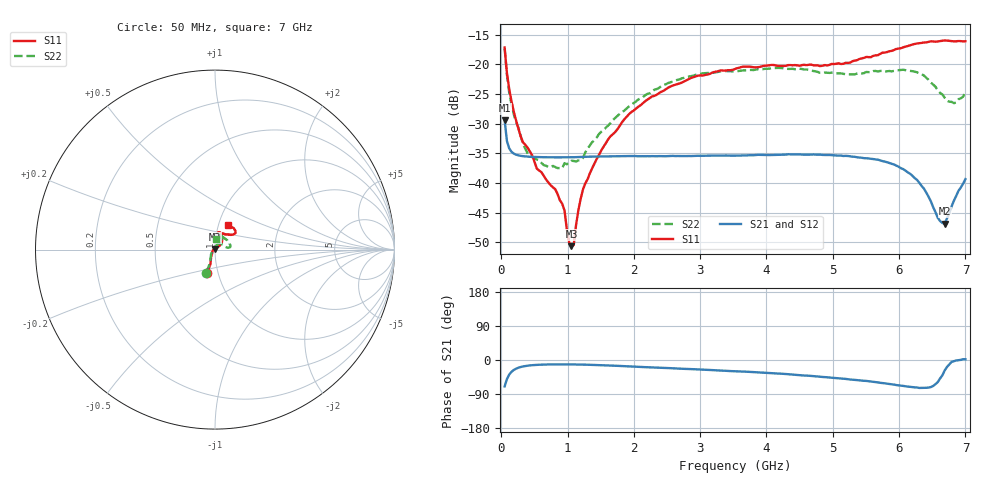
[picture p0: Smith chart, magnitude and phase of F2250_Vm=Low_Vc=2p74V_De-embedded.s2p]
! Integrated Device Technology
! Corporate Headquarters
! 6024 Silver Creek Valley Road
! San Jose, CA 95138  USA
! Phone:  1-408-284-8200
! Toll Free:  1-800-223-1366
! Webpage:  http://www.idt.com/
! Timing and RF Division
! 515 Groton Road, Suite 102
! Westford, MA 01886-6024
! Device:  F2250
! Description: Voltage Variable RF Attenuator
! Frequency:  50.0 -  6000.00 MHz
! Package:  3x3 mm Thin QFN Plastic Package: 16 pin
! Ports:  2 RF, 3 DC
!  Pin  1  = GND
!  Pin  2  = NC
!  Pin  3  = RF1  = Port 1
!  Pin  4  = NC
!  Pin  5  = GND
!  Pin  6  = GND
!  Pin  7  = GND
!  Pin  8  = GND
!  Pin  9  = NC
!  Pin 10  = RF2  = Port 2
!  Pin 11  = NC
!  Pin 12  = GND
!  Pin 13  = GND
!  Pin 14  = VCNTRL
!  Pin 15  = VDD
!  Pin 16  = VMODE
! Vcntrl:  2.740 Volts
! Vmode:  +0.000 Volts
! Vdd:  +3.30  Volts
! Current:  1.174 mA
! Data:  The device was measured on a the F2250 evaluation board which has
!  individual transmission lines to the RF pins.  Data was collected
!  using a calibrated network analyzer.  The evaluation board was
!  de-embedded using a TRL calibration technique.
!  The reference plane is the edge of the package pin.
! Misc:  SN 10
!  Action Tracker AT0258
! Date Measured:  2014-11-26
! Date:  2015-10-15  MJV
! Note:
!  Integrated Device Technology supplies this data as a sample of measured
!  data at the package pin for this product.  Your particular data for this
!  product may vary.
!  Data was taken at 25 degrees C.
!  Integrated Device Technology reserves the right to change this data at anytime.
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# GHz S dB R 50
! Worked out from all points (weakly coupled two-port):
!   201 points, 50 MHz to 7 GHz, reference 50 ohm
!   highest |S21| = -29.41 dB at 50 MHz (marker M1); lowest = -46.9 dB at 6.687 GHz (marker M2)
!   lowest |S11| = -50.6 dB at 1.058 GHz (marker M3), VSWR 1.01, Z = 49.8 + j0.245 ohm
!   |S11| at or under -10 dB: start of sweep to end of sweep
!   |S22| runs from -37.5 to -17.3 dB; largest |S21 - S12| = 6.5e-05
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0.05  -17.18 -108.6  -29.41 -69.8  -29.41 -69.8  -17.27 -111.0
0.08475  -21.45 -107.4  -32.92 -50.4  -32.92 -50.4  -21.75 -110.2
0.15425  -26.23 -116.6  -34.76 -31.2  -34.75 -31.1  -26.81 -122.5
0.29325  -32.20 -127.8  -35.43 -18.5  -35.43 -18.5  -32.09 -137.4
0.3975  -34.08 -141.7  -35.56 -15.0  -35.56 -15.0  -35.02 -160.3
0.5365  -37.59 -155.7  -35.63 -12.8  -35.64 -12.8  -36.06 178.0
0.91875  -43.49 157.8  -35.68 -11.5  -35.69 -11.5  -37.54 133.5
0.9535  -44.64 170.0  -35.69 -11.5  -35.68 -11.5  -36.65 131.0
1.023  -50.01 144.3  -35.68 -11.6  -35.67 -11.6  -36.63 116.0
1.05775  -50.65 123.2  -35.67 -11.6  -35.67 -11.6  -36.26 110.7
1.0925  -50.45 89.5  -35.66 -11.7  -35.65 -11.7  -36.29 106.5
1.162  -44.63 56.7  -35.64 -11.9  -35.64 -11.9  -36.21 95.5
1.2315  -41.10 44.2  -35.61 -12.1  -35.61 -12.1  -35.80 85.8
1.6485  -32.11 42.0  -35.52 -14.6  -35.51 -14.7  -29.88 64.5
2.37825  -24.86 47.3  -35.48 -20.3  -35.48 -20.3  -23.99 56.8
3.525  -20.79 72.4  -35.40 -29.5  -35.40 -29.5  -21.19 74.7
4.7065  -20.17 72.3  -35.20 -42.5  -35.20 -42.6  -21.14 72.3
5.85325  -17.82 40.5  -36.64 -63.3  -36.64 -63.3  -21.13 23.0
6.27025  -16.51 40.0  -39.49 -72.6  -39.50 -72.6  -21.36 9.7
6.68725  -15.99 48.7  -46.86 -27.7  -46.85 -27.4  -25.64 28.5
6.861  -16.13 55.1  -42.19 -1.3  -42.13 -1.3  -26.46 57.9
7  -16.13 63.2  -39.36 1.9  -39.31 1.7  -24.63 83.1
